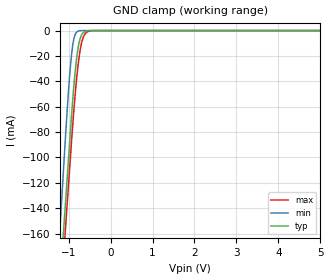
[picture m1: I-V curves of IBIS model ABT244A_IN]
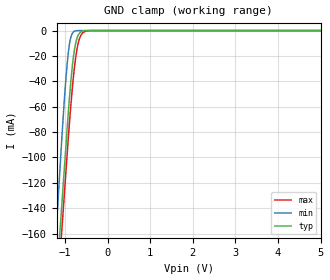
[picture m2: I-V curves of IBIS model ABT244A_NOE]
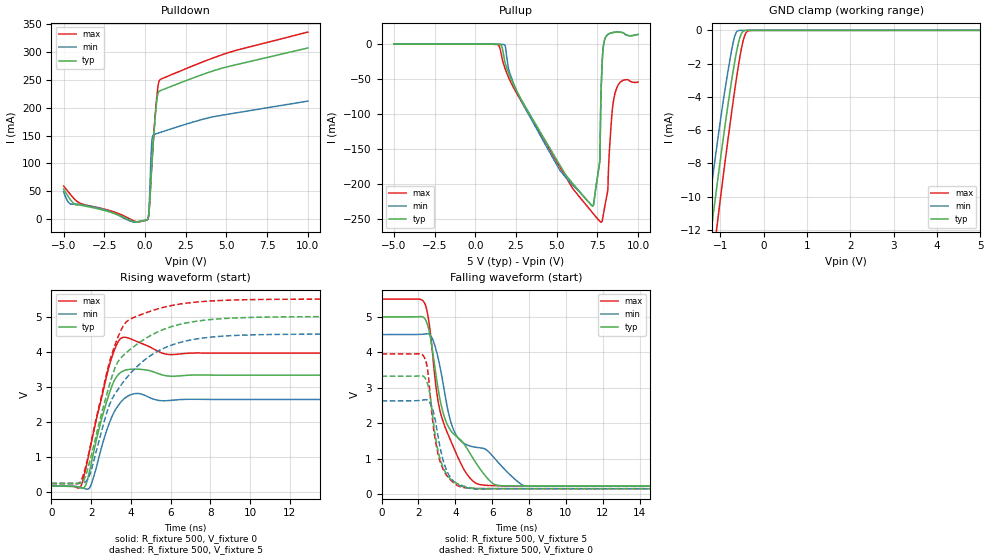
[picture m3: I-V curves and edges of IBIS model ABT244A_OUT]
| TEXAS INSTRUMENTS INCORPORATED
| Standard Linear and Logic Group
| IBIS Model of SN74ABT244A
| OCTAL BUFFERS/DRIVERS WITH 3-STATE OUTPUTS
| This file contains package information for the following:
|  SSOP 20-pin (DB) package as [Component] ABT244A_DB
|  SOIC 20-pin (DW) package as [Component] ABT244A_DW
|  PDIP 20-pin (N) package as [Component] ABT244A_N
|  TSSOP 20-pin (PW) package as [Component] ABT244A_PW
| This device can be powered at the following Vccs:
|  5 volt Vcc
| This file provides unique models under the [Model Selector] for each Vcc.
| For operation at a specific Vcc, select the appropriate model after each
| [Model Selector] keyword.
[IBIS Ver]   3.2
[Comment char]  |_char
[File Name]   sn74abt244a.ibs
[File Rev]   1.1 | h_die
[Date]   December 20, 2004
[Source]   Data created from TI-SPICE simulations at TI-SLL.
[Notes]   The following is an IBIS list for the ABT244A.
   Please contact sllibis@ti.com with questions and
   comments concerning SLL IBIS models.
   This IBIS model is created from a BA (back annotated netlist)
   - FILE REV HISTORY
   - 1.1 Release IBIS file on 12/20/04
   - Non-monotonic data and Decreassing Current warning in pullup
   and pulldown is due to resistor at output.
   - Power clamp data deleted as there is no power-clamp diode.
[Disclaimer] Property of Texas Instruments Incorporated.  Unauthorized
   reproduction and/or distribution is strictly prohibited.
   This product is protected under copyright law.
   Created  2004, (C) Copyright  2004, Texas Instruments
   Incorporated, All Rights Reserved
   UNLESS THERE IS A SIGNED, WRITTEN AGREEMENT TO THE
   CONTRARY, TEXAS INSTRUMENTS (TI) IS PROVIDING THE IBIS
   MODELS  AND WITHOUT ANY WARRANTY, EXPRESSED OR
   IMPLIED.  TI assumes no liability for:
   1) the accuracy of the IBIS models provided to your
   company;
   2) the proper functioning of these IBIS Models in your
   design or for any resulting applications; or
   3) infringement of patents, copyrights or intellectual
   property rights resulting from your use of these IBIS
   models.
   TI provides IBIS Models as a service to our customers.
   You and your company shall not distribute, sell or give
   these models to anyone else without prior written
   permission from TI.
   TI reserves the right to make changes to our products or
   to discontinue any semiconductor product or service
   without notice, and advises our customers to obtain the
   latest version of relevant information to verify, before
   placing orders, that the information being relied on is
   current.
   Please be aware that your receipt and use of the IBIS
   information provided shall serve as acceptance of these
   terms and conditions.  If you do not accept these terms,
   you should return or destroy the IBIS models and any
   other accompanying information immediately.
| Component ABT244A_DB 20-pin SSOP
[Component]   ABT244A_DB
[Manufacturer]   Texas Instruments, Inc.
[Package]
|   typ   min   max
R_pkg   4.000e-02   3.500e-02   5.100e-02
L_pkg   3.495e-09   3.035e-09   4.314e-09
C_pkg   4.200e-13   3.460e-13   5.020e-13
[Pin]   signal_name   model_name   R_pin   L_pin   C_pin
1   1NOE   ABT244A_NOE   4.900e-02   4.310e-09   5.020e-13
2   1A1   ABT244A_IN   4.800e-02   3.903e-09   4.870e-13
3   2Y4   ABT244A_OUT   3.500e-02   3.189e-09   3.960e-13
4   1A2   ABT244A_IN   3.500e-02   3.036e-09   3.470e-13
5   2Y3   ABT244A_OUT   3.500e-02   3.035e-09   3.670e-13
6   1A3   ABT244A_IN   3.500e-02   3.035e-09   3.670e-13
7   2Y2   ABT244A_OUT   3.500e-02   3.036e-09   3.470e-13
8   1A4   ABT244A_IN   3.500e-02   3.189e-09   3.970e-13
9   2Y1   ABT244A_OUT   4.700e-02   3.899e-09   4.880e-13
10   GND   GND   5.100e-02   4.314e-09   5.000e-13
11   2A1   ABT244A_IN   5.100e-02   4.314e-09   5.000e-13
12   1Y4   ABT244A_OUT   4.700e-02   3.899e-09   4.880e-13
13   2A2   ABT244A_IN   3.500e-02   3.189e-09   3.970e-13
14   1Y3   ABT244A_OUT   3.500e-02   3.036e-09   3.460e-13
15   2A3   ABT244A_IN   3.500e-02   3.035e-09   3.670e-13
16   1Y2   ABT244A_OUT   3.500e-02   3.035e-09   3.670e-13
17   2A4   ABT244A_IN   3.500e-02   3.036e-09   3.460e-13
18   1Y1   ABT244A_OUT   3.500e-02   3.189e-09   3.970e-13
19   2NOE   ABT244A_NOE   4.700e-02   3.899e-09   4.880e-13
20   VCC   POWER   5.100e-02   4.314e-09   5.020e-13
| Component ABT244A_DW 20-pin SOIC
[Component]   ABT244A_DW
[Manufacturer]   Texas Instruments, Inc.
[Package]
|   typ   min   max
R_pkg   3.800e-02   3.300e-02   4.500e-02
L_pkg   5.012e-09   4.110e-09   6.349e-09
C_pkg   7.170e-13   5.300e-13   8.680e-13
[Pin]   signal_name   model_name   R_pin   L_pin   C_pin
1   1NOE   ABT244A_NOE   4.200e-02   6.336e-09   8.650e-13
2   1A1   ABT244A_IN   4.300e-02   5.542e-09   8.670e-13
3   2Y4   ABT244A_OUT   3.400e-02   4.714e-09   7.320e-13
4   1A2   ABT244A_IN   3.400e-02   4.377e-09   5.910e-13
5   2Y3   ABT244A_OUT   3.600e-02   4.130e-09   5.330e-13
6   1A3   ABT244A_IN   3.500e-02   4.111e-09   5.300e-13
7   2Y2   ABT244A_OUT   3.400e-02   4.284e-09   5.830e-13
8   1A4   ABT244A_IN   3.400e-02   4.634e-09   7.260e-13
9   2Y1   ABT244A_OUT   4.000e-02   5.518e-09   8.650e-13
10   GND   GND   4.300e-02   6.349e-09   8.660e-13
11   2A1   ABT244A_IN   4.100e-02   6.281e-09   8.610e-13
12   1Y4   ABT244A_OUT   4.500e-02   5.561e-09   8.680e-13
13   2A2   ABT244A_IN   3.300e-02   4.778e-09   7.420e-13
14   1Y3   ABT244A_OUT   3.500e-02   4.414e-09   5.960e-13
15   2A3   ABT244A_IN   3.500e-02   4.110e-09   5.330e-13
16   1Y2   ABT244A_OUT   3.600e-02   4.130e-09   5.330e-13
17   2A4   ABT244A_IN   3.400e-02   4.377e-09   5.910e-13
18   1Y1   ABT244A_OUT   3.400e-02   4.714e-09   7.310e-13
19   2NOE   ABT244A_NOE   4.300e-02   5.569e-09   8.680e-13
20   VCC   POWER   4.200e-02   6.308e-09   8.640e-13
| Component ABT244A_N 20-pin PDIP
[Component]   ABT244A_N
[Manufacturer]   Texas Instruments, Inc.
[Package]
|   typ   min   max
R_pkg   4.300e-02   3.800e-02   5.000e-02
L_pkg   7.384e-09   4.680e-09   1.032e-08
C_pkg   5.100e-13   2.310e-13   8.210e-13
[Pin]   signal_name   model_name   R_pin   L_pin   C_pin
1   1NOE   ABT244A_NOE   4.200e-02   9.427e-09   8.100e-13
2   1A1   ABT244A_IN   4.600e-02   8.544e-09   4.560e-13
3   2Y4   ABT244A_OUT   4.800e-02   7.163e-09   4.350e-13
4   1A2   ABT244A_IN   4.000e-02   4.825e-09   2.610e-13
5   2Y3   ABT244A_OUT   4.000e-02   5.284e-09   6.480e-13
6   1A3   ABT244A_IN   4.000e-02   4.686e-09   2.320e-13
7   2Y2   ABT244A_OUT   4.000e-02   6.359e-09   4.890e-13
8   1A4   ABT244A_IN   3.800e-02   7.982e-09   4.750e-13
9   2Y1   ABT244A_OUT   4.300e-02   9.403e-09   4.750e-13
10   GND   GND   5.000e-02   1.032e-08   8.050e-13
11   2A1   ABT244A_IN   5.000e-02   1.028e-08   8.100e-13
12   1Y4   ABT244A_OUT   4.300e-02   9.383e-09   4.770e-13
13   2A2   ABT244A_IN   3.800e-02   7.978e-09   4.760e-13
14   1Y3   ABT244A_OUT   4.000e-02   6.302e-09   4.920e-13
15   2A3   ABT244A_IN   4.000e-02   4.680e-09   2.310e-13
16   1Y2   ABT244A_OUT   4.000e-02   5.284e-09   6.480e-13
17   2A4   ABT244A_IN   4.000e-02   4.822e-09   2.610e-13
18   1Y1   ABT244A_OUT   4.700e-02   7.118e-09   4.390e-13
19   2NOE   ABT244A_NOE   4.600e-02   8.492e-09   4.610e-13
20   VCC   POWER   4.300e-02   9.348e-09   8.210e-13
| Component ABT244A_PW 20-pin TSSOP
[Component]   ABT244A_PW
[Manufacturer]   Texas Instruments, Inc.
[Package]
|   typ   min   max
R_pkg   4.500e-02   3.600e-02   5.700e-02
L_pkg   2.694e-09   2.290e-09   3.177e-09
C_pkg   1.560e-13   7.600e-14   2.590e-13
[Pin]   signal_name   model_name   R_pin   L_pin   C_pin
1   1NOE   ABT244A_NOE   3.600e-02   3.045e-09   2.590e-13
2   1A1   ABT244A_IN   5.100e-02   3.013e-09   1.890e-13
3   2Y4   ABT244A_OUT   4.400e-02   2.695e-09   1.640e-13
4   1A2   ABT244A_IN   4.700e-02   2.362e-09   7.900e-14
5   2Y3   ABT244A_OUT   4.700e-02   2.333e-09   8.600e-14
6   1A3   ABT244A_IN   4.700e-02   2.298e-09   8.500e-14
7   2Y2   ABT244A_OUT   4.700e-02   2.351e-09   7.900e-14
8   1A4   ABT244A_IN   4.400e-02   2.706e-09   1.650e-13
9   2Y1   ABT244A_OUT   4.900e-02   2.999e-09   1.880e-13
10   GND   GND   3.900e-02   3.039e-09   2.570e-13
11   2A1   ABT244A_IN   3.800e-02   3.044e-09   2.580e-13
12   1Y4   ABT244A_OUT   5.700e-02   3.177e-09   1.990e-13
13   2A2   ABT244A_IN   4.400e-02   2.825e-09   1.730e-13
14   1Y3   ABT244A_OUT   4.700e-02   2.429e-09   8.300e-14
15   2A3   ABT244A_IN   4.900e-02   2.383e-09   9.000e-14
16   1Y2   ABT244A_OUT   4.900e-02   2.347e-09   8.900e-14
17   2A4   ABT244A_IN   4.700e-02   2.290e-09   7.600e-14
18   1Y1   ABT244A_OUT   4.500e-02   2.613e-09   1.580e-13
19   2NOE   ABT244A_NOE   4.400e-02   2.883e-09   1.810e-13
20   VCC   POWER   3.900e-02   3.044e-09   2.560e-13
| Models and submodels in the file (3): ABT244A_IN (Input), ABT244A_NOE (Input), ABT244A_OUT (3-state)
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[Model]   ABT244A_IN
Model_type  Input
Vinl=0.8
Vinh=2.0
| variable   typ   min   max
C_comp   2.98pF   2.25pF   4.56pF
[Temperature Range]   40   -40   100
| Ambient temperature   25   -40   85
[Voltage range]   5   4.5   5.5
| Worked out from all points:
|   GND clamp passes 1 mA (typ) near -0.62 V on its own axis
[GND Clamp]
| ABT244A_IN
|   Voltage   I(typ)   I(min)   I(max)
-5V       -2.023A    -2.247A    -2.022A
-1.855V   -511.9mA   -514.4mA   -527.5mA
-1.075V   -137mA     -84.7mA    -156.8mA
-1V       -100.9mA   -46.9mA    -121.2mA
-925mV    -65.25mA   -17.85mA   -85.55mA
-900mV    -54.4mA    -11.35mA   -74.27mA
-850mV    -35.11mA   -3.716mA   -53.41mA
-775mV    -14.29mA   -457.6uA   -27.94mA
-725mV    -6.493mA   -67.43uA   -15.76mA
-650mV    -1.652mA   -2.017uA   -5.335mA
-475mV    -17.97uA   -673.5pA   -221.3uA
5V        34.17pA    24.48pA    478.5pA
[Model]   ABT244A_NOE
Model_type  Input
Vinl=0.8
Vinh=2.0
| variable   typ   min   max
C_comp   2.89pF   2.22pF   4.35pF
[Temperature Range]   40   -40   100
| Ambient temperature   25   -40   85
[Voltage range]   5   4.5   5.5
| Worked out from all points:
|   GND clamp passes 1 mA (typ) near -0.62 V on its own axis
[GND Clamp]
| ABT244A_NOE
|   Voltage   I(typ)   I(min)   I(max)
-5V       -2.023A    -2.247A    -2.022A
-1.855V   -511.9mA   -514.4mA   -527.5mA
-1.075V   -137mA     -84.7mA    -156.8mA
-1V       -100.9mA   -46.9mA    -121.2mA
-925mV    -65.25mA   -17.85mA   -85.55mA
-900mV    -54.4mA    -11.35mA   -74.27mA
-850mV    -35.11mA   -3.716mA   -53.41mA
-775mV    -14.29mA   -457.6uA   -27.94mA
-725mV    -6.493mA   -67.43uA   -15.76mA
-650mV    -1.652mA   -2.017uA   -5.335mA
-475mV    -17.97uA   -673.5pA   -221.3uA
5V        34.17pA    24.48pA    478.5pA
[Model]   ABT244A_OUT
Model_type  3-state
Enable   Active-Low
Vref =   0
Rref =   500
Cref =   50p
Vmeas =   1.5
| variable   typ   min   max
C_comp   3.58pF   2.59pF   5.44pF
| C_pullup   3.81pF   2.58pF   6.31pF
| C_pulldown   6.83pF   0.59pF   27.80pF
| C_tri-state   3.58pF   2.59pF   5.44pF
[Temperature Range]   40   -40   100
| Ambient temperature   25   -40   85
[Voltage range]   5   4.5   5.5
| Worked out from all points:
|   slope of the pulldown table from 0 to 0.75 V, typ, clamps not added: 3.4 ohm
|   GND clamp passes 1 mA (typ) near -0.60 V on its own axis
|   rising waveform, R_fixture 500, V_fixture 0: 20-80 % time 852ps typ, 802ps min, 906ps max; typ from 0.157 V to 3.33 V
|   falling waveform, R_fixture 500, V_fixture 5: 20-80 % time 1.99ns typ, 2.87ns min, 1.27ns max; typ from 5 V to 0.234 V
|   rising waveform, R_fixture 500, V_fixture 5: 20-80 % time 1.86ns typ, 2.23ns min, 1.42ns max; typ from 0.234 V to 5 V
|   falling waveform, R_fixture 500, V_fixture 0: 20-80 % time 654ps typ, 655ps min, 615ps max; typ from 3.33 V to 0.157 V
[GND Clamp]
| ABT244A_OUT
|   Voltage   I(typ)   I(min)   I(max)
-5V       -127.4mA   -120.5mA   -133.6mA
-1.39V    -15.79mA   -13.22mA   -18.63mA
-1.305V   -13.98mA   -11.41mA   -16.73mA
-1.23V    -12.4mA    -9.86mA    -15.06mA
-1.15V    -10.74mA   -8.258mA   -13.31mA
-1.075V   -9.226mA   -6.805mA   -11.68mA
-730mV    -2.822mA   -1.032mA   -4.704mA
-650mV    -1.588mA   -201.3uA   -3.236mA
-580mV    -711.6uA   -11.99uA   -2.047mA
-445mV    -21.2uA    -21.08nA   -349.9uA
-305mV    -147.5nA   -179.9pA   -7.074uA
5V        432.9pA    568pA      3.844nA
[Pulldown]
| ABT244A_OUT
|   Voltage   I(typ)   I(min)   I(max)
-5V       54.05mA    49.64mA    59.37mA
-4.67V    38.56mA    29.25mA    47.56mA
-4.24V    25.71mA    27.32mA    33.55mA
-715mV    -4.025mA   -5.093mA   -2.507mA
125mV     -1.169mA   -743uA     -1.35mA
240mV     11.17mA    13.44mA    12.47mA
370mV     72.14mA    114.7mA    74.48mA
440mV     107.1mA    145.2mA    109.1mA
705mV     207.7mA    153.3mA    213.6mA
900mV     229.8mA    155.2mA    249.4mA
5.09V     273.4mA    188.1mA    298.3mA
10V       306.9mA    211.7mA    335.4mA
[Pullup]
| ABT244A_OUT
|   Voltage   I(typ)   I(min)   I(max)
-5V       -35.32pA   -25.92pA   -27.91pA
1.355V    -85.16uA   -694nA     -421.2uA
1.805V    -23.07mA   -738.6uA   -33.02mA
3.11V     -90.28mA   -93.01mA   -92.87mA
7.225V    -231mA     -231mA     -241.3mA
7.655V    -165.5mA   -165.5mA   -252.8mA
7.76V     -46.96mA   -46.96mA   -254.1mA
7.935V    5.194mA    5.194mA    -234.6mA
8.145V    13.79mA    13.79mA    -208.1mA
8.385V    16.3mA     16.3mA     -103.2mA
8.595V    17.15mA    17.15mA    -69.29mA
10V       13.9mA     13.9mA     -54.08mA
[Ramp]
| ABT244A_OUT
| variable   typ   min   max
dV/dt_r   2.04/9.29E-10   1.64/9.20E-10   2.58/1.04E-09
dV/dt_f   2.86/2.00E-09   2.58/2.87E-09   3.16/1.27E-09
R_load = 500
[Rising Waveform]
| ABT244A_OUT
R_fixture =   500
C_fixture =   0
L_fixture =   0
V_fixture =   0
V_fixture_min = 0
V_fixture_max = 0
|   Time   V(typ)   V(min)   V(max)
0s        157.4mV    154.9mV    155.8mV
1.495ns   101.3mV    114.2mV    166.2mV
1.725ns   183.7mV    76.68mV    646.3mV
1.98ns    732.5mV    169.7mV    1.317V
2.92ns    2.81V      1.962V     3.607V
3.3ns     3.293V     2.405V     4.212V
3.59ns    3.438V     2.614V     4.403V
4.335ns   3.496V     2.804V     4.281V
5.98ns    3.297V     2.604V     3.914V
24.99ns   3.327V     2.633V     3.955V
[Falling Waveform]
| ABT244A_OUT
R_fixture =   500
C_fixture =   0
L_fixture =   0
V_fixture =   5
V_fixture_min = 4.5
V_fixture_max = 5.5
|   Time   V(typ)   V(min)   V(max)
0s        5V         4.5V       5.5V
2.325ns   4.962V     4.513V     5.396V
2.77ns    4.02V      4.369V     3.942V
3.005ns   3.176V     3.976V     2.822V
3.255ns   2.468V     3.36V      2.183V
3.975ns   1.665V     1.74V      1.238V
5.19ns    830mV      1.318V     293.7mV
6.145ns   271.9mV    1.006V     240.6mV
7.89ns    234.1mV    228.4mV    233mV
24.99ns   234.1mV    227.8mV    232.2mV
[Rising Waveform]
| ABT244A_OUT
R_fixture =   500
C_fixture =   0
L_fixture =   0
V_fixture =   5
V_fixture_min = 4.5
V_fixture_max = 5.5
|   Time   V(typ)   V(min)   V(max)
0s        234.1mV    227.8mV    232.2mV
1.485ns   245.3mV    236.5mV    302.1mV
1.925ns   854.2mV    468.3mV    1.208V
2.805ns   2.809V     2.285V     3.432V
3.245ns   3.591V     2.826V     4.255V
3.75ns    3.957V     3.226V     4.834V
4.625ns   4.332V     3.73V      5.079V
6.265ns   4.748V     4.226V     5.338V
8.66ns    4.943V     4.442V     5.463V
24.99ns   5V         4.5V       5.5V
[Falling Waveform]
| ABT244A_OUT
R_fixture =   500
C_fixture =   0
L_fixture =   0
V_fixture =   0
V_fixture_min = 0
V_fixture_max = 0
|   Time   V(typ)   V(min)   V(max)
0s        3.327V     2.633V     3.955V
2.3ns     3.313V     2.66V      3.877V
2.51ns    3.08V      2.645V     3.461V
2.74ns    2.343V     2.439V     2.219V
2.915ns   1.646V     2.082V     1.528V
3.13ns    1.086V     1.445V     1.005V
3.345ns   749.7mV    948mV      698.8mV
3.605ns   509.5mV    589mV      481.2mV
4.31ns    259.4mV    229.9mV    203.9mV
24.99ns   157.4mV    154.9mV    155.9mV
